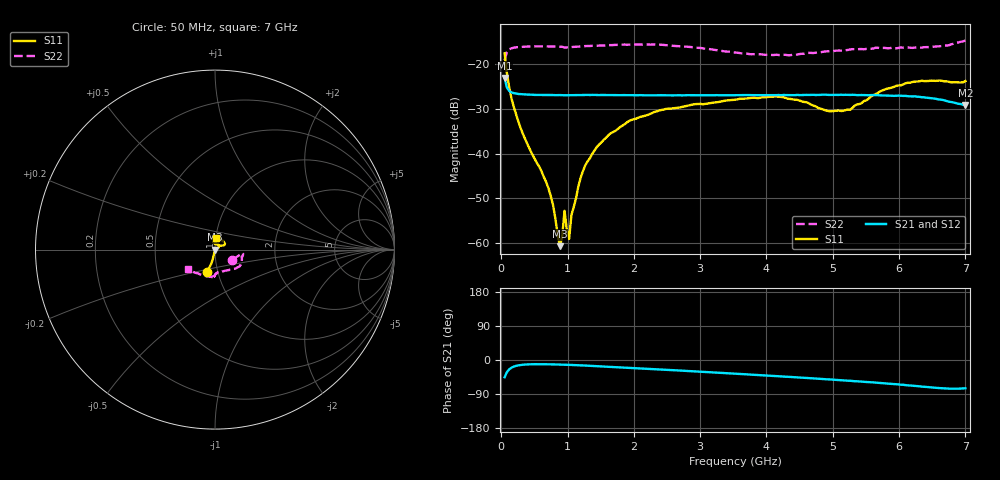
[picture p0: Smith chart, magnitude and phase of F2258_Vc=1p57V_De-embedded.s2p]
! Integrated Device Technology
! Corporate Headquarters
! 6024 Silver Creek Valley Road
! San Jose, CA 95138  USA
! Phone:  1-408-284-8200
! Toll Free:  1-800-223-1366
! Webpage:  http://www.idt.com/
! Timing and RF Division
! 515 Groton Road, Suite 102
! Westford, MA 01886-6024
! Device:  F2258
! Description: Voltage Variable RF Attenuator
! Frequency:  50.0 -  6000.00 MHz
! Package:  3x3 mm Thin QFN Plastic Package: 16 pin
! Ports:  2 RF, 2 DC
!  Pin  1  = NC
!  Pin  2  = NC
!  Pin  3  = RF2  = Port 2
!  Pin  4  = GND
!  Pin  5  = Vdd
!  Pin  6  = NC
!  Pin  7  = VCTRL
!  Pin  8  = NC
!  Pin  9  = GND
!  Pin 10  = RF1  = Port 1
!  Pin 11  = NC
!  Pin 12  = NC
!  Pin 13  = NC
!  Pin 14  = NC
!  Pin 15  = NC
!  Pin 16  = NC
! Vcntrl:  1.570 Volts
! Vdd:  +3.300 Volts
! Current:  1.161 mA
! Data:  The device was measured on a the F2258 evaluation board which has
!  individual transmission lines to the RF pins.  Data was collected
!  using a calibrated network analyzer.  The evaluation board was
!  de-embedded using a TRL calibration technique.
!  The reference plane is the edge of the package pin.
! Misc:  SN 10
!  Action Tracker AT0285
! Date Measured:  2014-12-10
! Date:  2016-01-13  MJV
! Note:
!  Integrated Device Technology supplies this data as a sample of measured
!  data at the package pin for this product.  Your particular data for this
!  product may vary.
!  Data was taken at 25 degrees C.
!  Integrated Device Technology reserves the right to change this data at anytime.
!Freq_(GHz)  S11M_(dB)  S11P_(deg)  S21M_(dB)  S21P_(deg)  S12M_(dB)  S12P_(deg)  S22M_(dB)  S22P_(deg)
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# GHz S dB R 50
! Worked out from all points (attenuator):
!   201 points, 50 MHz to 7 GHz, reference 50 ohm
!   highest |S21| = -23.08 dB at 50 MHz (marker M1); lowest = -29.1 dB at 7 GHz (marker M2)
!   lowest |S11| = -60.7 dB at 884 MHz (marker M3), VSWR 1.00, Z = 50.1 - j0.0307 ohm
!   |S11| at or under -10 dB: start of sweep to end of sweep
!   |S22| runs from -19.1 to -14.7 dB; largest |S21 - S12| = 0.00036
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0.05  -17.56 -109.1  -23.08 -45.4  -23.10 -45.4  -19.11 -29.9
0.1195  -25.19 -103.2  -25.97 -24.6  -25.98 -24.6  -16.66 -10.0
0.189  -29.58 -103.6  -26.46 -17.4  -26.50 -17.4  -16.29 -7.6
0.328  -35.64 -103.6  -26.72 -12.5  -26.73 -12.4  -16.09 -7.7
0.71025  -47.68 -94.5  -26.87 -11.3  -26.86 -11.3  -16.02 -11.7
0.77975  -51.43 -90.3  -26.88 -11.6  -26.89 -11.6  -16.02 -12.9
0.884  -60.68 -19.4  -26.89 -12.1  -26.90 -12.1  -16.07 -14.8
0.91875  -58.51 16.6  -26.92 -12.3  -26.89 -12.3  -16.08 -15.5
0.9535  -52.77 -108.9  -26.93 -12.5  -26.89 -12.5  -16.25 -15.2
0.98825  -57.07 -109.5  -26.93 -12.7  -26.88 -12.7  -16.24 -16.1
1.023  -59.06 -41.9  -26.89 -12.9  -26.89 -12.9  -16.17 -16.7
1.05775  -53.72 -12.3  -26.90 -13.1  -26.89 -13.1  -16.14 -17.0
1.2315  -43.91 17.2  -26.88 -14.4  -26.85 -14.4  -15.97 -19.6
1.44  -38.53 19.5  -26.87 -16.4  -26.88 -16.4  -15.86 -22.5
1.6485  -35.45 22.8  -26.87 -18.3  -26.85 -18.3  -15.72 -25.4
2.37825  -30.36 41.9  -26.93 -24.9  -26.94 -24.9  -15.63 -34.9
3.525  -27.93 88.7  -26.92 -36.1  -26.93 -36.1  -17.37 -57.7
4.1505  -27.21 103.8  -26.90 -42.6  -26.89 -42.6  -17.86 -76.4
4.7065  -29.21 94.1  -26.83 -48.5  -26.81 -48.5  -17.48 -87.4
5.2625  -30.17 49.9  -26.85 -54.8  -26.87 -54.8  -16.69 -91.4
5.85325  -25.35 27.0  -27.02 -62.6  -26.99 -62.6  -16.41 -93.4
7  -23.77 83.6  -29.12 -74.5  -29.12 -74.5  -14.67 -143.9
